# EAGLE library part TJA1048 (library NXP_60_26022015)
Dual high-speed CAN transceiver with Standby mode The TJA1048 is a dual high-speed CAN transceiver that provides an interface between a Controller Area Network (CAN) protocol controller and the physical two-wire CAN bus. The transceiver is designed for high-speed (up to 1 Mbit/s) CAN applications in the automotive industry, providing the differential transmit and receive capability to (a microcontroller with) a CAN protocol controller. The TJA1048 belongs to the third generation of high-speed CAN transceivers from NXP Semiconductors, offering significant improvements over first- and second-generation devices such as the TJA1040. It offers improved Electro Magnetic Compatibility (EMC) and ElectroStatic Discharge (ESD) performance, and also features: Ideal passive behavior to the CAN bus when the supply voltage is off A very low-current Standby mode with bus wake-up capability on both channels TJA1048T can be interfaced directly to microcontrollers with supply voltages from 3 V to 5 V These features make the TJA1048 an excellent choice for all types of HS-CAN networks containing more than one HS-CAN interface that require a low-power mode with wake-up capability via the CAN bus, especially for Body Control and Gateway units. AAL Eindhoven MK
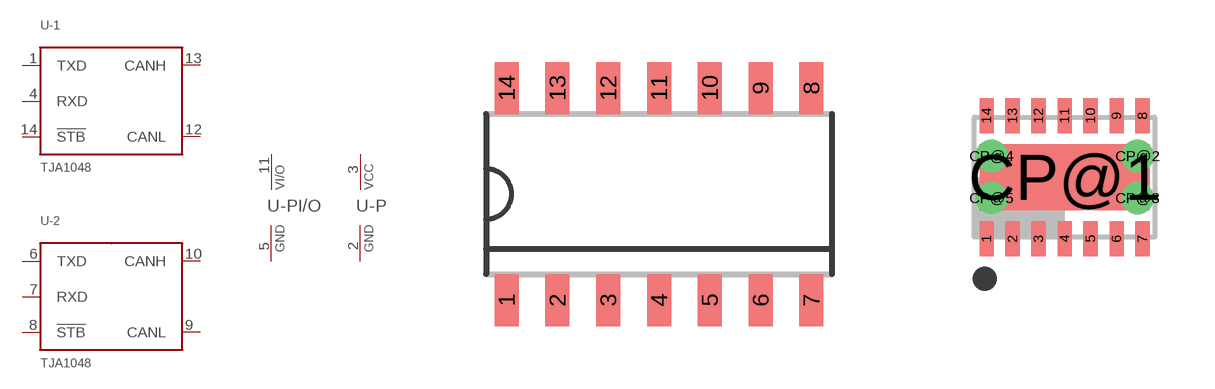
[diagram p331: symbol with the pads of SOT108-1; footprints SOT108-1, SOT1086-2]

Designator prefix U; gates -1=TJA1048 -2=TJA1048 -PI/O=PWRN-2 -P=PWRN

## TJA1048T  [SOT108-1]
1  -1:TXD  out
2  -P:GND  pwr
3  -P:VCC  pwr
4  -1:RXD
5  -PI/O:GND  pwr
6  -2:TXD  out
7  -2:RXD
8  -2:!STB  pas
9  -2:CANL
10  -2:CANH
11  -PI/O:VI/O  pwr
12  -1:CANL
13  -1:CANH
14  -1:!STB  pas

## TJA1048TK  [SOT1086-2]
1  -1:TXD  out
2  -P:GND  pwr
3  -P:VCC  pwr
4  -1:RXD
5  -PI/O:GND  pwr
6  -2:TXD  out
7  -2:RXD
8  -2:!STB  pas
9  -2:CANL
10  -2:CANH
11  -PI/O:VI/O  pwr
12  -1:CANL
13  -1:CANH
14  -1:!STB  pas
CP@1  -P:GND  pwr
CP@2  -P:GND  pwr
CP@3  -P:GND  pwr
CP@4  -P:GND  pwr
CP@5  -P:GND  pwr

## Footprint SOT108-1 (pad centres in mm)
SOT108-1 SO14: plastic small outline package; 14 leads; body width 3.9 mm; body thickness 1.47 mm JEDEC: MS-012 IEC: --
smd 0.6 x 1.3: 1 -3.81,-2.65; 2 -2.54,-2.65; 3 -1.27,-2.65; 4 0,-2.65; 5 1.27,-2.65; 6 2.54,-2.65; 7 3.81,-2.65; 8 3.81,2.65; 9 2.54,2.65; 10 1.27,2.65; 11 0,2.65; 12 -1.27,2.65; 13 -2.54,2.65; 14 -3.81,2.65

## Footprint SOT1086-2 (pad centres in mm)
SOT1086-2 HVSON14: plastic, thermal enhanced very thin small outline package; no leads; 14 terminals; body 3 x 4.5 x 0.85 mm JEDEC: MO-229 IEC: -- JEITA: -- ATTENTION: To be able to use this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
smd 0.35 x 0.875: 1 -1.95,-1.538; 2 -1.3,-1.538; 3 -0.65,-1.538; 4 0,-1.538; 5 0.65,-1.538; 6 1.3,-1.538; 7 1.95,-1.538; 8 1.95,1.538; 9 1.3,1.538; 10 0.65,1.538; 11 0,1.538; 12 -0.65,1.538; 13 -1.3,1.538; 14 -1.95,1.538
smd 4.25 x 1.65: CP@1 0,0
drill 0.3 pad 0.6: CP@2 1.825,0.525; CP@3 1.825,-0.525; CP@4 -1.825,0.525; CP@5 -1.825,-0.525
